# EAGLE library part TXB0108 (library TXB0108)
8-Bit Bi-Directional Level Shifter 1.2V-3.6V (VCCA) to 1.65V-5.5V (VCCB) bi-directional level shifter with auto direction sensing. Max data rate - VCCA 1.8V: 20Mbps (50ns), VCCA 3.3V: 100Mbps (10ns) Digikey: 296-21527-1-ND
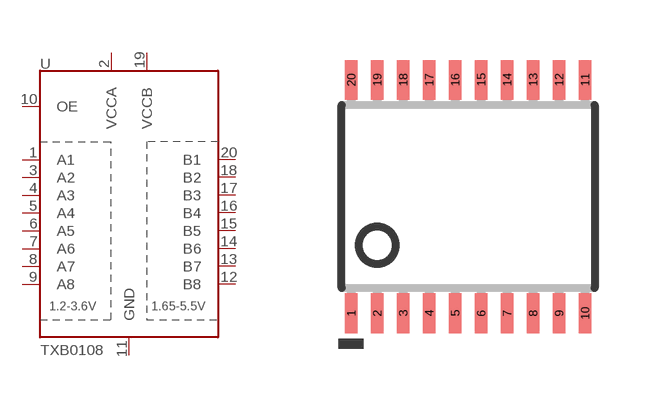
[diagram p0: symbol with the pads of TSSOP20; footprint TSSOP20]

Designator prefix U

## TXB0108 (Availability: Unavailable; Description: 8-Bit Bidirectional Voltage-Level Translator with Auto Direction Sensing and +/-15-kV ESD Protect; MF: Texas Instruments; MP: TXB0108; Package: None; Price: None)  [TSSOP20]
1  A1
2  VCCA
3  A2
4  A3
5  A4
6  A5
7  A6
8  A7
9  A8
10  OE
11  GND
12  B8
13  B7
14  B6
15  B5
16  B4
17  B3
18  B2
19  VCCB
20  B1

## Footprint TSSOP20 (pad centres in mm)
smd 0.305 x 0.991: 1 -2.925,-2.918; 2 -2.275,-2.918; 3 -1.625,-2.918; 4 -0.975,-2.918; 5 -0.325,-2.918; 6 0.325,-2.918; 7 0.975,-2.918; 8 1.625,-2.918; 9 2.275,-2.918; 10 2.925,-2.918; 11 2.925,2.918; 12 2.275,2.918; 13 1.625,2.918; 14 0.975,2.918; 15 0.325,2.918; 16 -0.325,2.918; 17 -0.975,2.918; 18 -1.625,2.918; 19 -2.275,2.918; 20 -2.925,2.918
